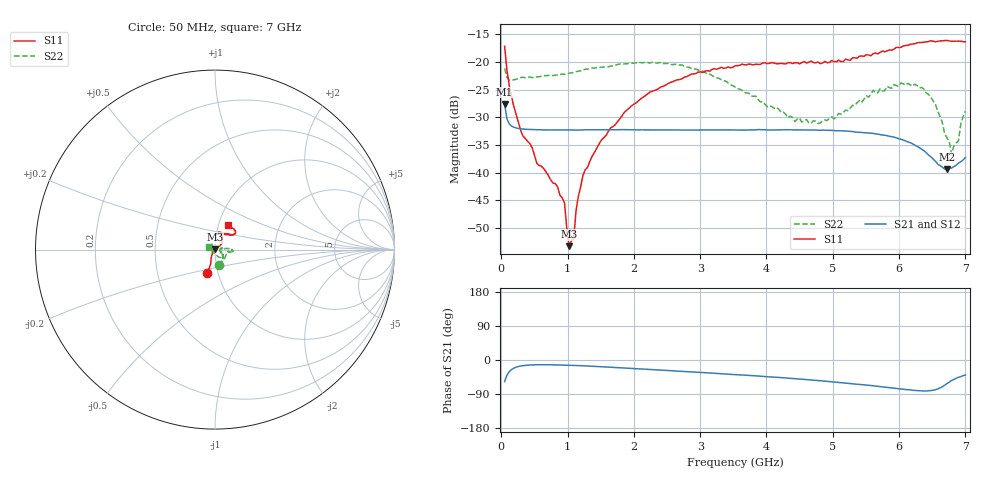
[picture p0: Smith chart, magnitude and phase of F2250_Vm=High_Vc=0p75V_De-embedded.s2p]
! Integrated Device Technology
! Corporate Headquarters
! 6024 Silver Creek Valley Road
! San Jose, CA 95138  USA
! Phone:  1-408-284-8200
! Toll Free:  1-800-223-1366
! Webpage:  http://www.idt.com/
! Timing and RF Division
! 515 Groton Road, Suite 102
! Westford, MA 01886-6024
! Device:  F2250
! Description: Voltage Variable RF Attenuator
! Frequency:  50.0 -  6000.00 MHz
! Package:  3x3 mm Thin QFN Plastic Package: 16 pin
! Ports:  2 RF, 3 DC
!  Pin  1  = GND
!  Pin  2  = NC
!  Pin  3  = RF1  = Port 1
!  Pin  4  = NC
!  Pin  5  = GND
!  Pin  6  = GND
!  Pin  7  = GND
!  Pin  8  = GND
!  Pin  9  = NC
!  Pin 10  = RF2  = Port 2
!  Pin 11  = NC
!  Pin 12  = GND
!  Pin 13  = GND
!  Pin 14  = VCNTRL
!  Pin 15  = VDD
!  Pin 16  = VMODE
! Vcntrl:  0.750 Volts
! Vmode:  +3.300 Volts
! Vdd:  +3.30  Volts
! Current:  1.296 mA
! Data:  The device was measured on a the F2250 evaluation board which has
!  individual transmission lines to the RF pins.  Data was collected
!  using a calibrated network analyzer.  The evaluation board was
!  de-embedded using a TRL calibration technique.
!  The reference plane is the edge of the package pin.
! Misc:  SN 10
!  Action Tracker AT0258
! Date Measured:  2014-11-26
! Date:  2015-10-15  MJV
! Note:
!  Integrated Device Technology supplies this data as a sample of measured
!  data at the package pin for this product.  Your particular data for this
!  product may vary.
!  Data was taken at 25 degrees C.
!  Integrated Device Technology reserves the right to change this data at anytime.
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# GHz S dB R 50
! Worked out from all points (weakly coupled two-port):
!   201 points, 50 MHz to 7 GHz, reference 50 ohm
!   highest |S21| = -27.60 dB at 50 MHz (marker M1); lowest = -39.4 dB at 6.722 GHz (marker M2)
!   lowest |S11| = -53.3 dB at 1.023 GHz (marker M3), VSWR 1.00, Z = 49.9 + j0.157 ohm
!   |S11| at or under -10 dB: start of sweep to end of sweep
!   |S22| runs from -36.7 to -20.1 dB; largest |S21 - S12| = 8.7e-05
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0.05  -17.15 -107.9  -27.60 -57.1  -27.60 -57.1  -21.15 -77.0
0.1195  -24.20 -111.1  -31.18 -30.8  -31.17 -30.8  -23.26 -28.7
0.29325  -32.39 -125.7  -32.09 -15.8  -32.09 -15.8  -22.81 -13.1
0.9535  -45.45 172.5  -32.30 -13.5  -32.28 -13.5  -22.26 -9.9
1.023  -53.28 133.4  -32.30 -13.9  -32.30 -13.9  -22.03 -9.7
1.0925  -51.86 72.4  -32.30 -14.3  -32.29 -14.3  -21.92 -9.7
1.12725  -46.86 51.1  -32.29 -14.5  -32.29 -14.5  -21.75 -10.2
1.2315  -40.52 36.2  -32.27 -15.3  -32.26 -15.3  -21.42 -11.2
1.6485  -31.93 39.5  -32.26 -19.1  -32.23 -19.1  -20.76 -9.3
2.37825  -24.75 45.9  -32.29 -26.4  -32.28 -26.4  -20.12 -4.8
3.525  -20.70 71.3  -32.30 -38.4  -32.32 -38.4  -24.53 5.3
4.4285  -20.16 74.4  -32.25 -49.3  -32.25 -49.3  -30.77 7.7
4.7065  -20.12 71.7  -32.28 -53.3  -32.29 -53.2  -30.62 -3.5
5.01925  -19.95 63.1  -32.39 -58.1  -32.39 -58.2  -30.25 -14.0
5.85325  -17.82 40.3  -33.42 -72.8  -33.42 -73.0  -24.65 -38.5
6.3745  -16.43 40.7  -36.02 -81.7  -36.03 -81.8  -24.91 -53.2
6.54825  -16.37 44.5  -37.94 -78.4  -37.97 -78.4  -27.66 -67.9
6.722  -16.12 49.1  -39.37 -62.0  -39.37 -62.0  -33.68 -103.1
6.7915  -16.28 51.1  -39.17 -54.1  -39.15 -54.2  -36.66 -130.9
6.89575  -16.24 56.2  -38.27 -45.5  -38.23 -45.8  -34.24 179.4
6.9305  -16.26 58.5  -38.03 -43.8  -38.01 -43.9  -31.17 170.0
7  -16.37 62.2  -37.27 -39.7  -37.24 -40.0  -28.90 159.7
